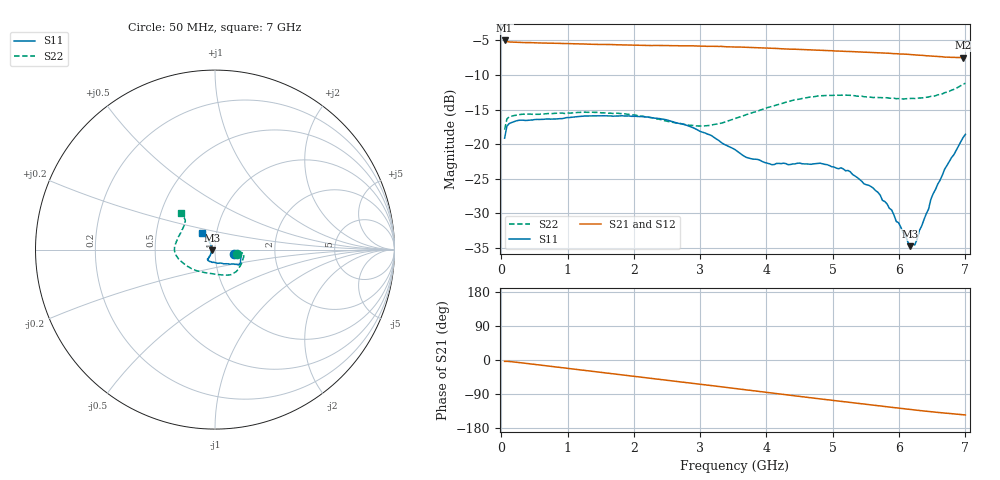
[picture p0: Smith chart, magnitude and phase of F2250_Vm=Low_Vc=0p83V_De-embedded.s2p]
! Integrated Device Technology
! Corporate Headquarters
! 6024 Silver Creek Valley Road
! San Jose, CA 95138  USA
! Phone:  1-408-284-8200
! Toll Free:  1-800-223-1366
! Webpage:  http://www.idt.com/
! Timing and RF Division
! 515 Groton Road, Suite 102
! Westford, MA 01886-6024
! Device:  F2250
! Description: Voltage Variable RF Attenuator
! Frequency:  50.0 -  6000.00 MHz
! Package:  3x3 mm Thin QFN Plastic Package: 16 pin
! Ports:  2 RF, 3 DC
!  Pin  1  = GND
!  Pin  2  = NC
!  Pin  3  = RF1  = Port 1
!  Pin  4  = NC
!  Pin  5  = GND
!  Pin  6  = GND
!  Pin  7  = GND
!  Pin  8  = GND
!  Pin  9  = NC
!  Pin 10  = RF2  = Port 2
!  Pin 11  = NC
!  Pin 12  = GND
!  Pin 13  = GND
!  Pin 14  = VCNTRL
!  Pin 15  = VDD
!  Pin 16  = VMODE
! Vcntrl:  0.830 Volts
! Vmode:  +0.000 Volts
! Vdd:  +3.30  Volts
! Current:  1.168 mA
! Data:  The device was measured on a the F2250 evaluation board which has
!  individual transmission lines to the RF pins.  Data was collected
!  using a calibrated network analyzer.  The evaluation board was
!  de-embedded using a TRL calibration technique.
!  The reference plane is the edge of the package pin.
! Misc:  SN 10
!  Action Tracker AT0258
! Date Measured:  2014-11-26
! Date:  2015-10-15  MJV
! Note:
!  Integrated Device Technology supplies this data as a sample of measured
!  data at the package pin for this product.  Your particular data for this
!  product may vary.
!  Data was taken at 25 degrees C.
!  Integrated Device Technology reserves the right to change this data at anytime.
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# GHz S dB R 50
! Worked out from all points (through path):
!   201 points, 50 MHz to 7 GHz, reference 50 ohm
!   highest |S21| = -5.00 dB at 50 MHz (marker M1); lowest = -7.5 dB at 6.965 GHz (marker M2)
!   group delay of S21, straight-line fit = 58.1 ps
!   lowest |S11| = -34.8 dB at 6.166 GHz (marker M3), VSWR 1.04, Z = 48.2 - j0.317 ohm
!   |S11| at or under -10 dB: start of sweep to end of sweep
!   |S22| runs from -17.9 to -11.2 dB; largest |S21 - S12| = 0.0018
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0.05  -19.14 -11.8  -5.00 -3.6  -5.01 -3.6  -17.91 -10.8
0.08475  -17.39 -6.9  -5.17 -3.5  -5.16 -3.5  -16.35 -7.1
0.22375  -16.64 -7.1  -5.28 -5.8  -5.26 -5.8  -15.82 -9.8
1.2315  -15.96 -26.8  -5.50 -27.0  -5.49 -27.0  -15.38 -42.8
2.37825  -16.30 -33.2  -5.72 -50.6  -5.72 -50.6  -16.39 -70.0
3.0385  -18.29 -41.4  -5.82 -64.7  -5.81 -64.7  -17.39 -100.4
3.525  -20.79 -59.2  -5.95 -75.3  -5.95 -75.3  -16.29 -128.6
3.69875  -21.92 -69.5  -5.99 -79.0  -5.98 -79.1  -15.72 -137.3
4.081  -22.98 -94.1  -6.14 -87.3  -6.13 -87.3  -14.54 -154.1
4.7065  -22.86 -122.4  -6.39 -100.5  -6.39 -100.5  -13.15 -172.3
5.2625  -23.99 -127.5  -6.60 -112.0  -6.61 -112.0  -12.94 175.0
5.6795  -26.96 -128.4  -6.76 -120.6  -6.77 -120.6  -13.26 164.7
5.85325  -29.29 -133.1  -6.85 -124.1  -6.87 -124.1  -13.35 160.1
5.888  -29.53 -133.9  -6.89 -124.8  -6.88 -124.8  -13.35 159.5
5.9575  -31.19 -138.7  -6.91 -126.2  -6.92 -126.2  -13.42 157.1
6.166  -34.77 -169.6  -7.03 -130.5  -7.03 -130.5  -13.41 150.3
6.2355  -34.59 166.4  -7.08 -131.8  -7.07 -131.9  -13.40 147.8
6.444  -29.41 131.4  -7.23 -135.8  -7.22 -135.9  -13.19 141.3
6.5135  -27.19 127.3  -7.28 -137.1  -7.28 -137.1  -13.09 139.1
6.68725  -23.62 123.0  -7.41 -140.0  -7.41 -140.0  -12.55 135.1
6.96525  -19.05 127.6  -7.49 -144.5  -7.50 -144.5  -11.37 133.5
7  -18.58 127.8  -7.49 -145.0  -7.49 -145.1  -11.18 133.0
